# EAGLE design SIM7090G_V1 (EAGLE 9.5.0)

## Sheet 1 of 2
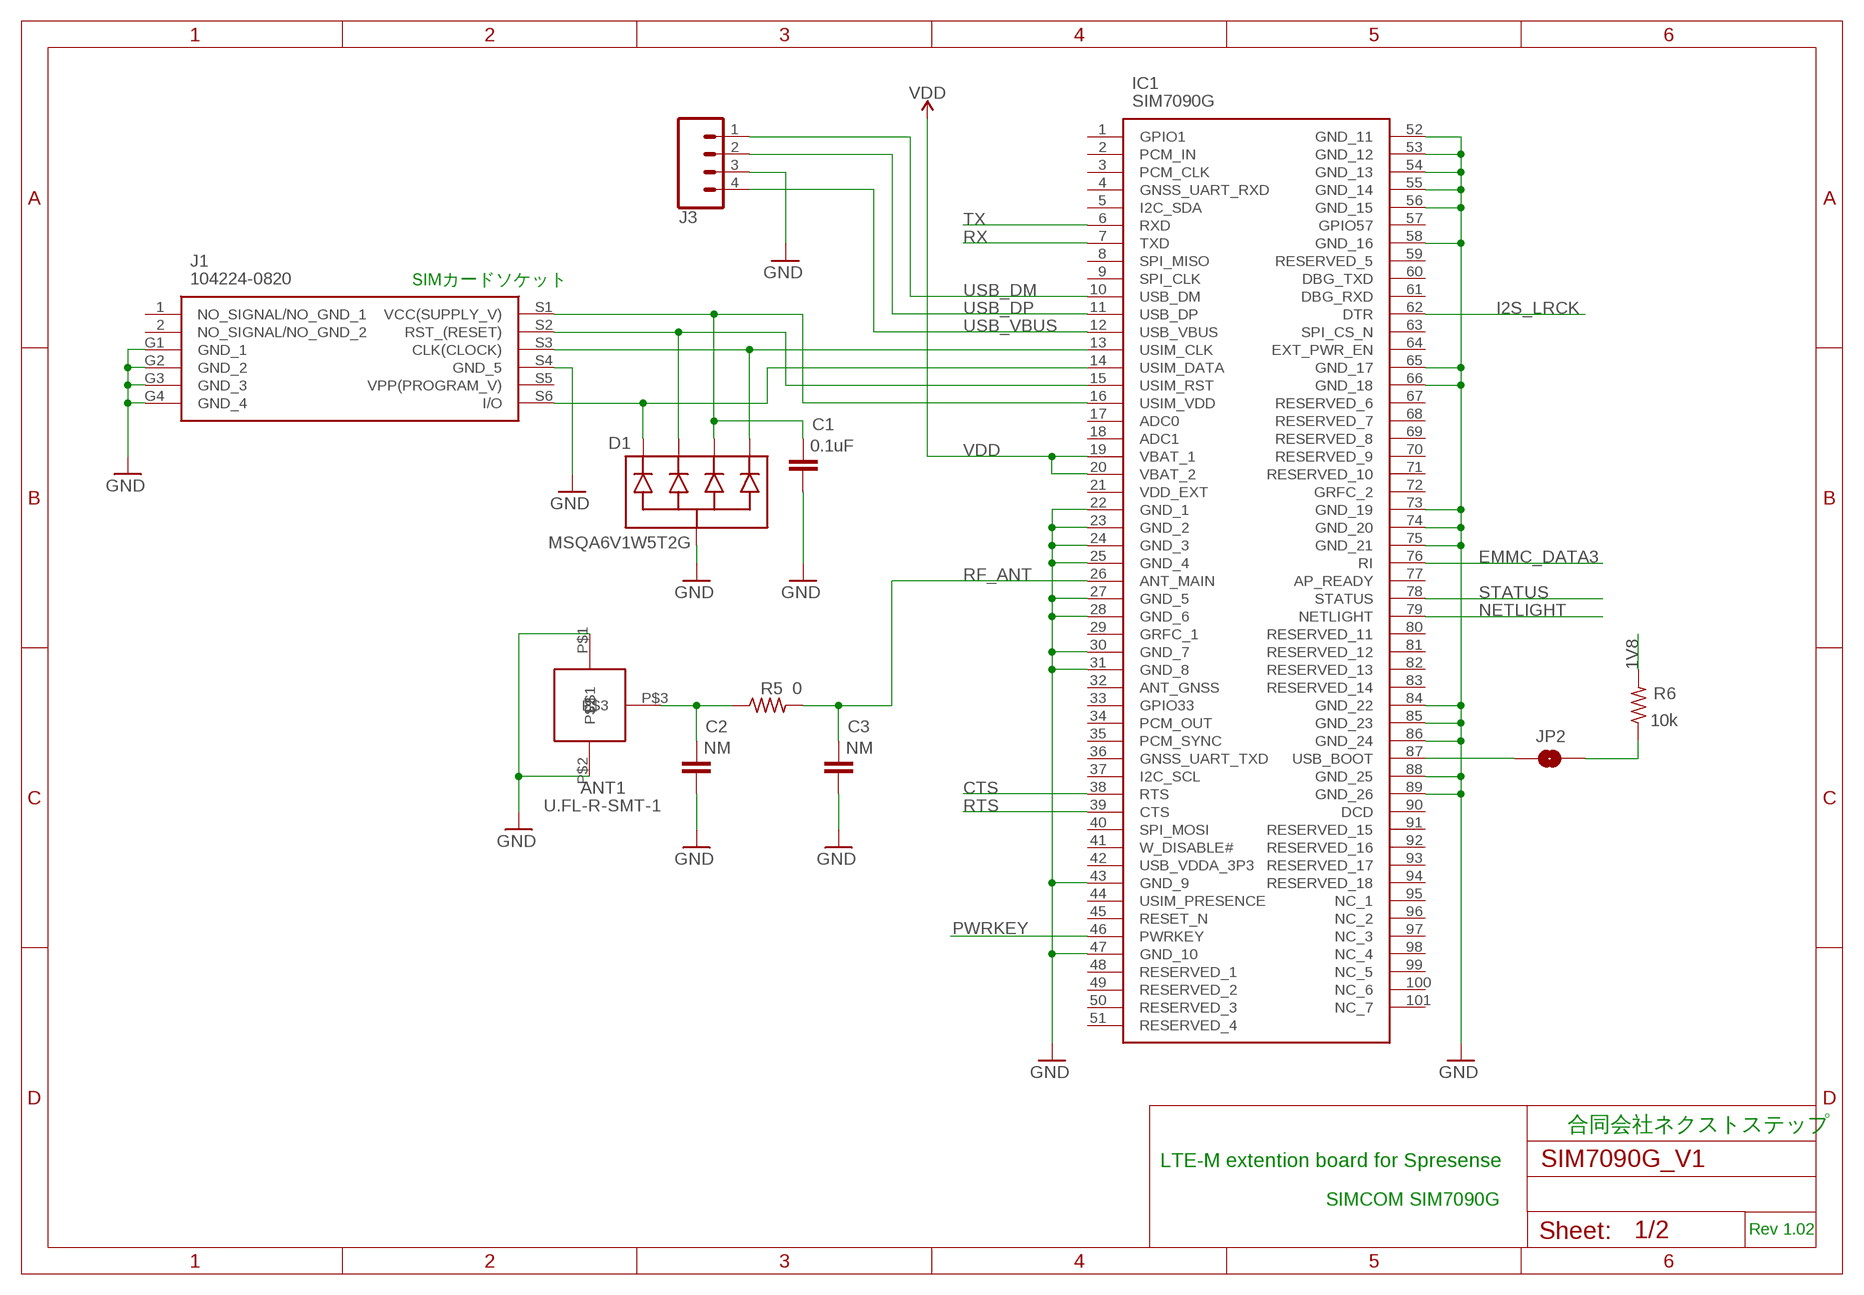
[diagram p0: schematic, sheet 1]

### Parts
ANT1  U.FL-R-SMT-1  [U.FL-R-SMT-1]
C1  0.1uF  C-EUC0603K  [C0603K]
C2  NM  C-EUC0603K  [C0603K]
C3  NM  C-EUC0603K  [C0603K]
D1  MSQA6V1W5T2G  TVS-DIODE-ARRAY-4X  [SOT-353]
IC1  SIM7090G  [SIM7090G]
J1  104224-0820  [1042240820]
J3  CONN_041.27MM  [1X04_1.27MM]
JP2  JUMPER-SMT_2_NO_NO-SILK  [SMT-JUMPER_2_NO_NO-SILK]
R5  0  R-US_R0603  [R0603]
R6  10k  R-US_R0603  [R0603]

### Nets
1V8: R6.2 ; also sheet 2
CTS: IC1.38(RTS) ; also sheet 2
EMMC_DATA3: IC1.76(RI) ; also sheet 2
GND: ANT1.P$1 ANT1.P$2 C1.2 C2.2 C3.2 D1.2(COM) IC1.22(GND_1) IC1.23(GND_2) IC1.24(GND_3) IC1.25(GND_4) IC1.27(GND_5) IC1.28(GND_6) IC1.30(GND_7) IC1.31(GND_8) IC1.43(GND_9) IC1.47(GND_10) IC1.52(GND_11) IC1.53(GND_12) IC1.54(GND_13) IC1.55(GND_14) IC1.56(GND_15) IC1.58(GND_16) IC1.65(GND_17) IC1.66(GND_18) IC1.73(GND_19) IC1.74(GND_20) IC1.75(GND_21) IC1.84(GND_22) IC1.85(GND_23) IC1.86(GND_24) IC1.88(GND_25) IC1.89(GND_26) J1.G1(GND_1) J1.G2(GND_2) J1.G3(GND_3) J1.G4(GND_4) J1.S4(GND_5) J3.3 ; also sheet 2
I2S_LRCK: IC1.62(DTR) ; also sheet 2
N$2: IC1.87(USB_BOOT) JP2.1
N$3: JP2.2 R6.1
N$4: ANT1.P$3 C2.1 R5.1
NETLIGHT: IC1.79(NETLIGHT) ; also sheet 2
PWRKEY: IC1.46(PWRKEY) ; also sheet 2
RF_ANT: C3.1 IC1.26(ANT_MAIN) R5.2
RTS: IC1.39(CTS) ; also sheet 2
RX: IC1.7(TXD) ; also sheet 2
SIM_CLK1: D1.1 IC1.13(USIM_CLK) J1.S3(CLK(CLOCK))
SIM_DATA1: D1.5 IC1.14(USIM_DATA) J1.S6(I/O)
SIM_RST1: D1.4 IC1.15(USIM_RST) J1.S2(RST_(RESET))
SIM_VCC1: C1.1 D1.3 IC1.16(USIM_VDD) J1.S1(VCC(SUPPLY_V))
STATUS: IC1.78(STATUS) ; also sheet 2
TX: IC1.6(RXD) ; also sheet 2
USB_DM: IC1.10(USB_DM) J3.1
USB_DP: IC1.11(USB_DP) J3.2
USB_VBUS: IC1.12(USB_VBUS) J3.4
VDD: IC1.19(VBAT_1) IC1.20(VBAT_2) ; also sheet 2
Unconnected: IC1.1(GPIO1) IC1.2(PCM_IN) IC1.3(PCM_CLK) IC1.4(GNSS_UART_RXD) IC1.5(I2C_SDA) IC1.8(SPI_MISO) IC1.9(SPI_CLK) IC1.17(ADC0) IC1.18(ADC1) IC1.21(VDD_EXT) IC1.29(GRFC_1) IC1.32(ANT_GNSS) IC1.33(GPIO33) IC1.34(PCM_OUT) IC1.35(PCM_SYNC) IC1.36(GNSS_UART_TXD) IC1.37(I2C_SCL) IC1.40(SPI_MOSI) IC1.41(W_DISABLE#) IC1.42(USB_VDDA_3P3) IC1.44(USIM_PRESENCE) IC1.45(RESET_N) IC1.48(RESERVED_1) IC1.49(RESERVED_2) IC1.50(RESERVED_3) IC1.51(RESERVED_4) IC1.57(GPIO57) IC1.59(RESERVED_5) IC1.60(DBG_TXD) IC1.61(DBG_RXD) IC1.63(SPI_CS_N) IC1.64(EXT_PWR_EN) IC1.67(RESERVED_6) IC1.68(RESERVED_7) IC1.69(RESERVED_8) IC1.70(RESERVED_9) IC1.71(RESERVED_10) IC1.72(GRFC_2) IC1.77(AP_READY) IC1.80(RESERVED_11) IC1.81(RESERVED_12) IC1.82(RESERVED_13) IC1.83(RESERVED_14) IC1.90(DCD) IC1.91(RESERVED_15) IC1.92(RESERVED_16) IC1.93(RESERVED_17) IC1.94(RESERVED_18) IC1.95(NC_1) IC1.96(NC_2) IC1.97(NC_3) IC1.98(NC_4) IC1.99(NC_5) IC1.100(NC_6) IC1.101(NC_7) J1.1(NO_SIGNAL/NO_GND_1) J1.2(NO_SIGNAL/NO_GND_2) J1.S5(VPP(PROGRAM_V))

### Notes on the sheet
- SIMカードソケット
- 合同会社ネクストステップ
- LTE-M extention board for Spresense
- SIMCOM SIM7090G
- Rev 1.02

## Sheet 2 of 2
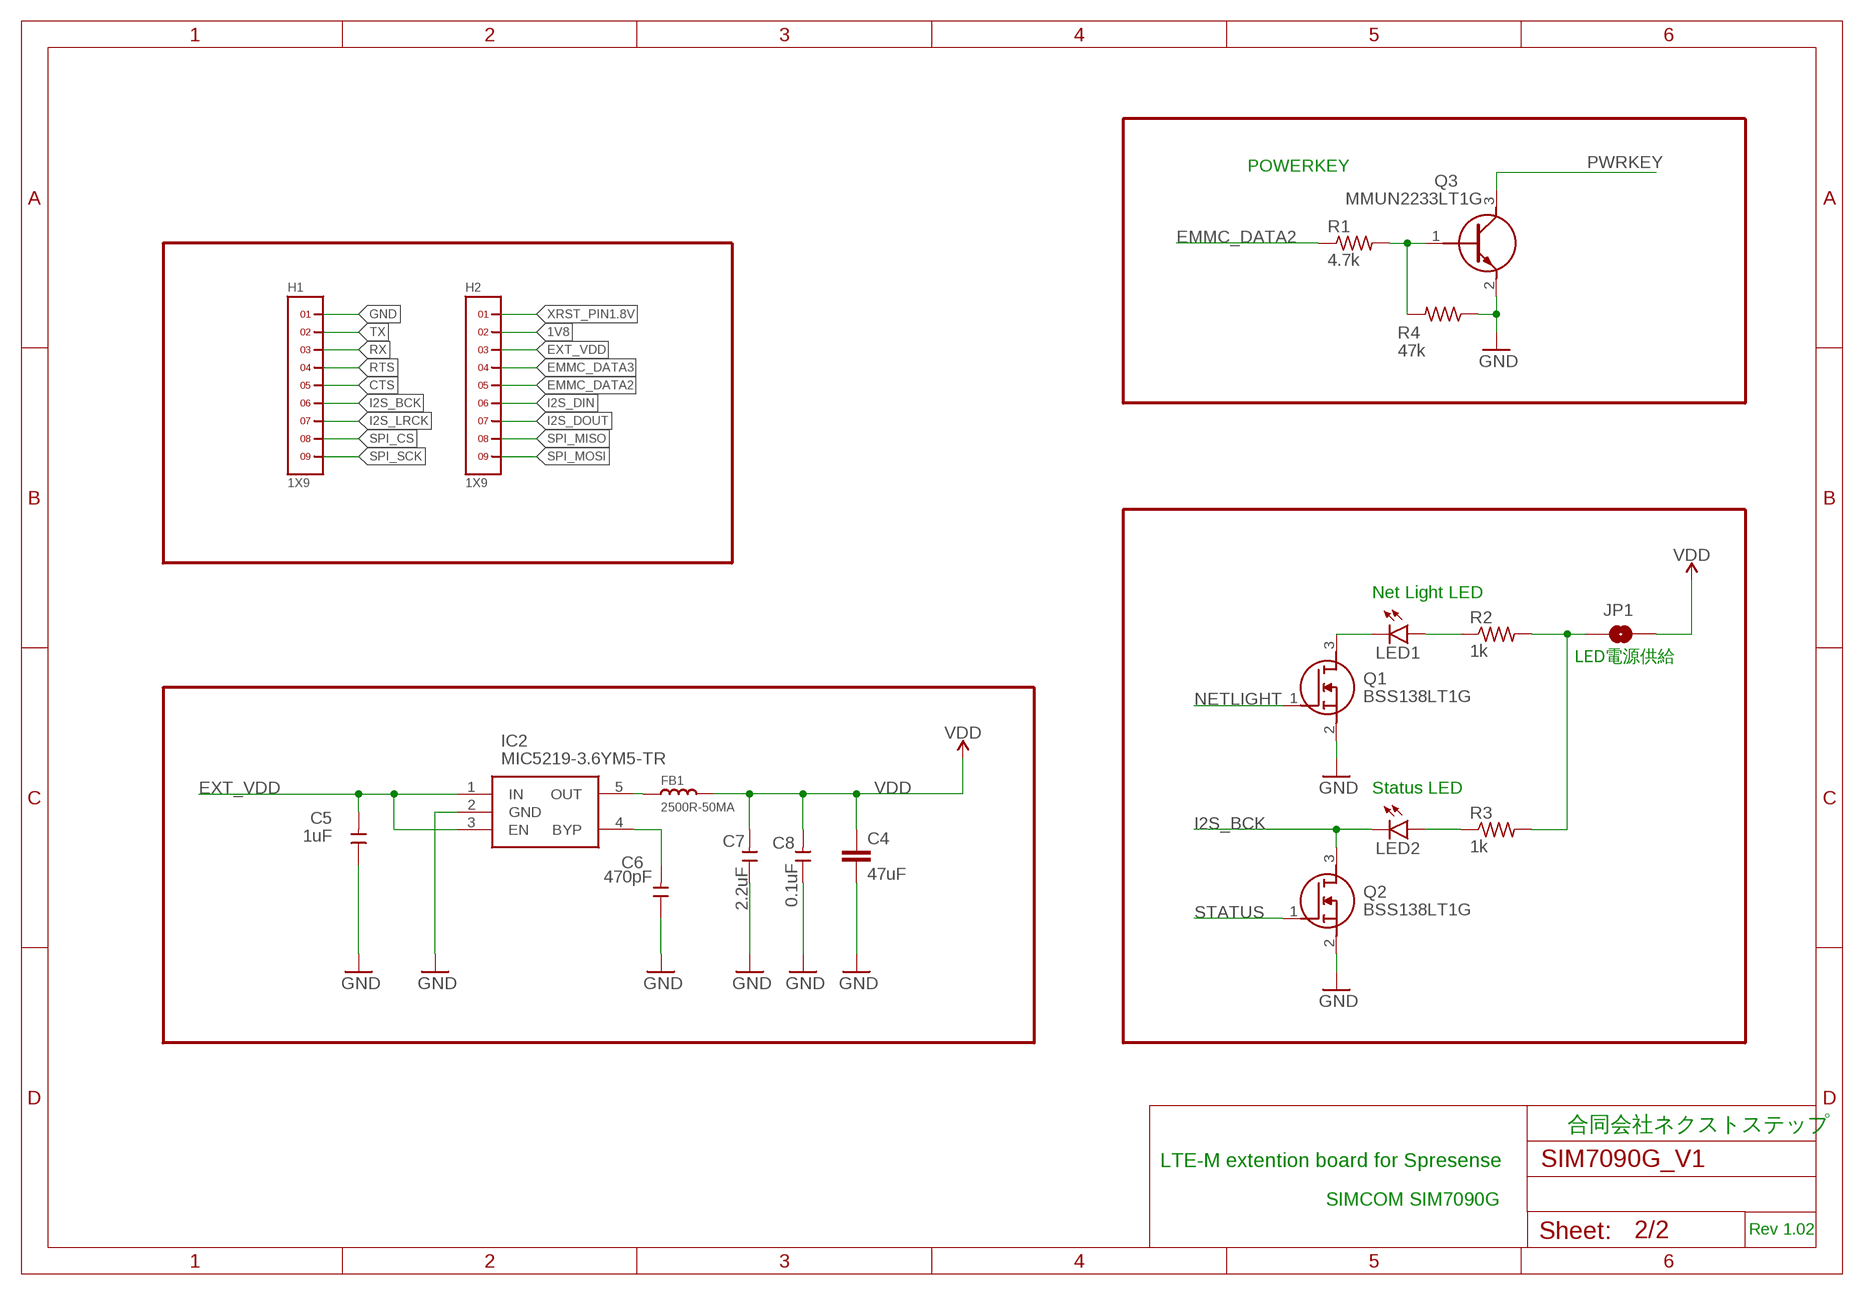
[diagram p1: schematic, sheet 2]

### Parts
C4  47uF  C-EUC0805  [C0805]
C5  1uF  CERAMIC-1UF-25V-10%-X7R(0603)  [C0603]
C6  470pF  CERAMIC-100NF-50V-10%-X7R(0603)  [C0603]
C7  2.2uF  CERAMIC-100NF-50V-10%-X7R(0603)  [C0603]
C8  0.1uF  CERAMIC-100NF-50V-10%-X7R(0603)  [C0603]
FB1  2500R-50MA  SMD-FERRITE-BEAD-2500R-50MA(0603)  [L0603]
H1  1X9  [1X9]
H2  1X9  [1X9]
IC2  MIC5219-3.6YM5-TR  [SOT95P280X145-5N]
JP1  JUMPER-SMT_2_NO_NO-SILK  [SMT-JUMPER_2_NO_NO-SILK]
LED1  LEDCHIP-LED0603  [CHIP-LED0603]
LED2  LEDCHIP-LED0603  [CHIP-LED0603]
Q1  BSS138LT1G  [SOT96P237X111-3N]
Q2  BSS138LT1G  [SOT96P237X111-3N]
Q3  MMUN2233LT1G  [SOT96P237X111-3N]
R1  4.7k  R-US_R0603  [R0603]
R2  1k  R-US_R0603  [R0603]
R3  1k  R-US_R0603  [R0603]
R4  47k  R-US_R0603  [R0603]

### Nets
1V8: H2.2 ; also sheet 1
CTS: H1.5 ; also sheet 1
EMMC_DATA2: H2.5 R1.1
EMMC_DATA3: H2.4 ; also sheet 1
EXT_VDD: C5.2 H2.3 IC2.1(IN) IC2.3(EN)
GND: C4.2 C5.1 C6.1 C7.1 C8.1 H1.1 IC2.2(GND) Q1.2(S) Q2.2(S) Q3.2(E) R4.1 ; also sheet 1
I2S_BCK: H1.6 LED2.C Q2.3(D)
I2S_DIN: H2.6
I2S_DOUT: H2.7
I2S_LRCK: H1.7 ; also sheet 1
N$1: FB1.1 IC2.5(OUT)
N$9: C6.2 IC2.4(BYP)
N$13: JP1.1 R2.2 R3.2
N$16: LED1.A R2.1
N$19: Q3.1(B) R1.2 R4.2
N$22: LED2.A R3.1
NETLIGHT: Q1.1(G) ; also sheet 1
NETLIGHT_MON: LED1.C Q1.3(D)
PWRKEY: Q3.3(C) ; also sheet 1
RTS: H1.4 ; also sheet 1
RX: H1.3 ; also sheet 1
SPI_CS: H1.8
SPI_MISO: H2.8
SPI_MOSI: H2.9
SPI_SCK: H1.9
STATUS: Q2.1(G) ; also sheet 1
TX: H1.2 ; also sheet 1
VDD: C4.1 C7.2 C8.2 FB1.2 JP1.2 ; also sheet 1
XRST_PIN1.8V: H2.1

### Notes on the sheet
- POWERKEY
- Net Light LED
- LED電源供給
- Status LED
- 合同会社ネクストステップ
- LTE-M extention board for Spresense
- SIMCOM SIM7090G
- Rev 1.02

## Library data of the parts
ANT1 = Kris:U.FL-R-SMT-1: U.FL-R-SMT-1
C1-C4 = rcl:C-EU: CAPACITOR, European symbol; SPICEPREFIX: C
C5 = Seeed-Capacitor:CERAMIC-1UF-25V-10%-X7R(0603): 302010139; MPN: CC0603KRX7R8BB105; VALUE: 1uf
C6-C8 = Seeed-Capacitor:CERAMIC-100NF-50V-10%-X7R(0603): 302010138; MPN: CC0603KRX7R9BB104; VALUE: 100nf
D1 = TimWoo-Diodes:TVS-DIODE-ARRAY-4X
FB1 = Seeed-Inductor:SMD-FERRITE-BEAD-2500R-50MA(0603): 303030020
H1 H2 = headers(.1in):1X9
IC1 = SIM7090G:SIM7090G: LPWA Module Source: Datasheet; DESCRIPTION: LPWA Module; HEIGHT: 2.05mm; MANUFACTURER_NAME: Sim Com; MANUFACTURER_PART_NUMBER: SIM7090G
IC2 = SamacSys_Parts:MIC5219-3.6YM5-TR: LDO Voltage Regulators 500mA Peak 1% Low Noise LDO Source: Datasheet; DESCRIPTION: LDO Voltage Regulators 500mA Peak 1% Low Noise LDO; HEIGHT: 1.45mm; MANUFACTURER_NAME: Microchip; MANUFACTURER_PART_NUMBER: MIC5219-3.6YM5-TR; MOUSER_PART_NUMBER: 998-MIC5219-3.6YM5TR; MOUSER_PRICE-STOCK: https://www.mouser.co.uk/ProductDetail/Microchip-Technology-Micrel/MIC5219-36YM5-TR/?qs=U6T8BxXiZAWOHIj15bI33A%3D%3D
J1 = SamacSys_Parts:104224-0820: Memory Card Connectors nanoSIM 1.11mm Card Conn 6Ckt Push/Pull Source: Datasheet; DESCRIPTION: Memory Card Connectors nanoSIM 1.11mm Card Conn 6Ckt Push/Pull; HEIGHT: 1.11mm; MANUFACTURER_NAME: Molex; MANUFACTURER_PART_NUMBER: 104224-0820; MOUSER_PART_NUMBER: 538-104224-0820; MOUSER_PRICE-STOCK: https://www.mouser.com/Search/Refine.aspx?Keyword=538-104224-0820
J3 = SparkFun-Connectors:CONN_04: Multi connection point. Often used as Generic Header-pin footprint for 0.1 inch spaced/style header connections On any of the 0.1 inch spaced packages, you can populate with these: Break Away Headers - Straight (PRT-00116) Break Away Male Headers - Right Angle (PRT-00553) Female Headers (PRT-00115)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
JP1 JP2 = SparkFun-Jumpers:JUMPER-SMT_2_NO: Normally open jumper
LED1 LED2 = led:LED: LED
Q1 Q2 = SamacSys_Parts:BSS138LT1G: MOSFET N-Channel 50V 0.2A SOT23 ON Semiconductor BSS138LT1G N-channel MOSFET Transistor, 0.2 A, 50 V, 3-Pin SOT-23 Source: Datasheet; DESCRIPTION: MOSFET N-Channel 50V 0.2A SOT23 ON Semiconductor BSS138LT1G N-channel MOSFET Transistor, 0.2 A, 50 V, 3-Pin SOT-23; HEIGHT: 1.11mm; MANUFACTURER_NAME: ON Semiconductor; MANUFACTURER_PART_NUMBER: BSS138LT1G; MOUSER_PART_NUMBER: 863-BSS138LT1G; MOUSER_PRICE-STOCK: https://www.mouser.com/Search/Refine.aspx?Keyword=863-BSS138LT1G
Q3 = SamacSys_Parts:MMUN2233LT1G: ON SEMICONDUCTOR - MMUN2233LT1G - TRANSISTOR, SMD NPN Source: Datasheet; DESCRIPTION: ON SEMICONDUCTOR - MMUN2233LT1G - TRANSISTOR, SMD NPN; HEIGHT: 1.11mm; MANUFACTURER_NAME: ON Semiconductor; MANUFACTURER_PART_NUMBER: MMUN2233LT1G; MOUSER_PART_NUMBER: 863-MMUN2233LT1G; MOUSER_PRICE-STOCK: https://www.mouser.com/Search/Refine.aspx?Keyword=863-MMUN2233LT1G
R1-R6 = rcl:R-US_: RESISTOR, American symbol; SPICEPREFIX: R

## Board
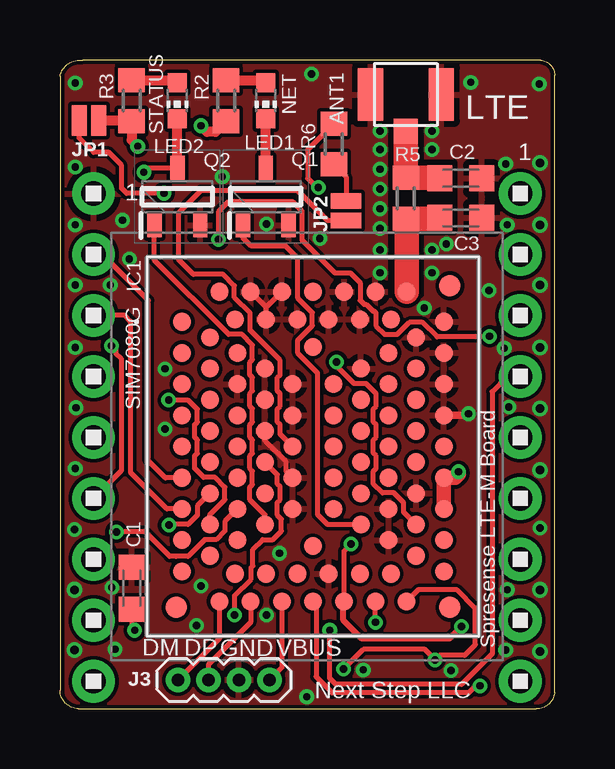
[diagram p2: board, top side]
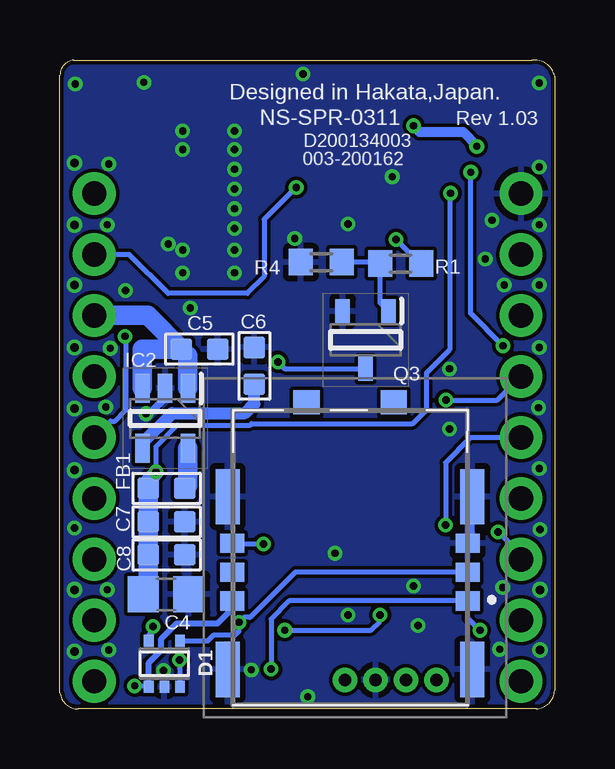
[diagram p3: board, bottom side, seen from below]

Size 20.61 x 27.03 mm. Coordinates in mm from the lower left corner, seen from the top.
Outline: 0,26.35 arc-88 0.95,27.02 20.03,27.02 arc-88 20.61,26.38 20.61,0.67 arc-88 19.84,0 0.76,0 arc-88 0,0.76 0,26.35
Copper layers (1*16): Top 0.035mm / dielectric 1.5mm / Bottom 0.035mm
Design rules "SeeedStudio_2layer_DRU_no_angle_20140221 *": minimum track width 6mil, minimum drill 12mil, track to track 6mil, track to pad 6mil, pad to pad 6mil, via to via 6mil, smd to smd 0mil, copper to edge 6mil, drill to drill 8mil, minimum pad ring 10mil, minimum via ring 6mil, stop-mask expansion 2mil, vias tented up to drill 100mil, thermal gap 10mil
tRestrict: 13 lines

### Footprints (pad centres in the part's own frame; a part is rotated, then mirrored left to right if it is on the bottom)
U.FL-R-SMT-1 = smd 1.05 x 2.2: P$1 -1.475,0; P$2 1.475,0 | smd 1 x 1.05: P$3 0,-1.525
C0603K = smd 1.05 x 1.08: 1 -0.875,0; 2 0.875,0
C0805 = smd 1.3 x 1.5: 1 -0.95,0; 2 0.95,0
C0603 = smd 0.889 x 0.889: 1 0,0.762; 2 0,-0.762
SOT-353 = smd 0.4 x 0.5: 1 -0.65,-0.95; 2 0,-0.95; 3 0.65,-0.95; 4 0.65,0.95; 5 -0.65,0.95
L0603 = smd 0.889 x 0.889: 1 -0.762,0; 2 0.762,0
1X9 = drill 1.016 pad 1.778: 1 0,0; 2 2.54,0; 3 5.08,0; 4 7.62,0; 5 10.16,0; 6 12.7,0; 7 15.24,0; 8 17.78,0; 9 20.32,0
SIM7090G = smd 0.75 x 0.75: 1 -5.45,5.2; 2 -5.45,3.9; 3 -5.45,2.6; 4 -5.45,1.3; 5 -5.45,0; 6 -5.45,-1.3; 7 -5.45,-2.6; 8 -5.45,-3.9; 9 -5.45,-5.2; 10 -3.9,-6.45; 11 -2.6,-6.45; 12 -1.3,-6.45; 13 0,-6.45; 14 1.3,-6.45; 15 2.6,-6.45; 16 3.9,-6.45; 17 5.45,-5.2; 18 5.45,-3.9; 19 5.45,-2.6; 20 5.45,-1.3; 21 5.45,0; 22 5.45,1.3; 23 5.45,2.6; 24 5.45,3.9; 25 5.45,5.2; 26 3.9,6.45; 27 2.6,6.45; 28 1.3,6.45; 29 0,6.45; 30 -1.3,6.45; 31 -2.6,6.45; 32 -3.9,6.45; 33 -4.3,4.55; 34 -4.3,3.25; 35 -4.3,1.95; 36 -4.3,0.65; 37 -4.3,-0.65; 38 -4.3,-1.95; 39 -4.3,-3.25; 40 -4.3,-4.55; 41 -1.95,-5.3; 42 -0.65,-5.3; 43 0.65,-5.3; 44 1.95,-5.3; 45 4.3,-4.55; 46 4.3,-3.25; 47 4.3,-1.95; 48 4.3,-0.65; 49 4.3,0.65; 50 4.3,1.95; 51 4.3,3.25; 52 4.3,4.55; 53 1.95,5.3; 54 0.65,5.3; 55 -0.65,5.3; 56 -1.95,5.3; 57 -3.15,3.9; 58 -3.15,2.6; 59 -3.15,1.3; 60 -3.15,0; 61 -3.15,-1.3; 62 -3.15,-2.6; 63 -3.15,-3.9; 64 0,-4.15; 65 3.15,-3.9; 66 3.15,-2.6; 67 3.15,-1.3; 68 3.15,0; 69 3.15,1.3; 70 3.15,2.6; 71 3.15,3.9; 72 0,4.15; 73 -2,3.25; 74 -2,1.95; 75 -2,0.65; 76 -2,-0.65; 77 -2,-1.95; 78 -2,-3.25; 79 2,-3.25; 80 2,-1.95; 81 2,-0.65; 82 2,0.65; 83 2,1.95; 84 2,3.25; 85 -0.85,2.6; 86 -0.85,1.3; 87 -0.85,0; 88 -0.85,-1.3; 89 -0.85,-2.6; 90 0.85,-2.6; 91 0.85,-1.3; 92 0.85,0; 93 0.85,1.3; 94 0.85,2.6; 95 -3.25,5.3; 96 -3.25,-5.3; 97 3.25,-5.3; 98 3.25,5.3 | smd 0.9 x 0.9: 99 -5.7,-6.7; 100 5.7,-6.7; 101 5.7,6.7
SOT95P280X145-5N = smd 1.2 x 0.6: 1 -1.25,0.95; 2 -1.25,0; 3 -1.25,-0.95; 4 1.25,-0.95; 5 1.25,0.95
1042240820 = smd 1.1 x 1: 1 -2.02,6.063; 2 1.62,6.063 | smd 1 x 2.3: G1 -5.3,-5.063; G2 -5.3,2.137; G3 4.9,2.137; G4 4.9,-5.063 | smd 1 x 0.8: S1 4.7,-2.212; S2 4.7,-1.012; S3 -5.1,-2.212; S4 4.7,0.188; S5 -5.1,-1.012; S6 -5.1,0.188
1X04_1.27MM = drill 0.508 pad 1: 1 0,0; 2 1.27,0; 3 2.54,0; 4 3.81,0
SMT-JUMPER_2_NO_NO-SILK = smd 0.635 x 1.27: 1 -0.406,0; 2 0.406,0
CHIP-LED0603 = smd 0.8 x 0.8: A 0,-0.75; C 0,0.75
SOT96P237X111-3N = smd 1 x 0.6: 1 -1.2,0.955; 2 -1.2,-0.955; 3 1.2,0
R0603 = smd 1 x 1.1: 1 -0.85,0; 2 0.85,0

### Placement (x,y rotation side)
ANT1  14.41,25.59 0 top
C1  2.98,5.02 90 top
C2  16.7,22.1 0 top
C3  16.7,20.45 0 top
C4  16.19,4.76 0 bottom
C5  14.8,14.99 270 bottom
C6  12.51,14.29 0 bottom
C7  16.16,7.78 270 bottom
C8  16.16,6.41 270 bottom
D1  16.26,1.87 0 bottom
FB1  16.16,9.18 180 bottom
H1  1.4,21.46 270 top
H2  19.18,21.46 270 top
IC1  10.54,10.92 0 top
IC2  16.22,12.1 270 bottom
J1  8.32,6.7 0 bottom
J3  4.92,1.2 0 top
JP1  1.21,24.51 180 top
JP2  11.93,20.75 90 top
LED1  8.57,25.34 180 top
LED2  4.89,25.34 180 top
Q1  8.57,21.34 90 top
Q2  4.89,21.34 90 top
Q3  7.87,15.37 270 bottom
R1  6.41,18.54 180 bottom
R2  6.92,25.34 270 top
R3  2.98,25.34 270 top
R4  9.72,18.61 0 bottom
R5  14.41,21.27 270 top
R6  11.41,23.53 90 top

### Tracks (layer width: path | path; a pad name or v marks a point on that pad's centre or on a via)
1V8  (via drill 0.3)
  Top 0.203: R6.2 10.32,23.28 10.32,22.1 10.7,21.72 v10.76,21.72
  Bottom 0.203: v10.76,21.72 12.1,20.38 12.1,18 12.79,17.3 16.1,17.3 17.72,18.92 H2.2
CTS  (via drill 0.3)
  Top 0.203: IC1.38 5.72,8.45 5.72,8.06 5.34,7.68 4.57,7.68 v4.54,7.65
  Bottom 0.203: v4.54,7.65 4.54,10.25 3.49,11.3 H1.5
EMMC_DATA2  (via drill 0.3)
  Top 0.203: v17.9,15.51 17.88,15.49 15.71,15.49 15.1,16.1 14.56,16.1 14.05,15.59 13.53,15.59 13.16,15.96 13.16,16.49 13.08,16.57 13.03,16.57 12.75,16.85 12.68,16.85 12.51,17.02 12.51,17.75 12.1,18.16 11.45,18.16 10.08,19.53 10.08,20.74 9.71,21.11 7.02,21.11 6.6,20.7 v6.6,19.55
  Bottom 0.203: H2.5 18.5,11.98 18.31,11.98 17.87,12.43 17.87,15.48 v17.9,15.51 | v6.6,19.55 5.6,18.54 R1.1
EMMC_DATA3  (via drill 0.3)
  Top 0.203: H2.4 18.64,13.84 18,13.21 18,2.29 16.73,1.02 11.49,1.02 11.24,1.27 v11.24,3.27 | v7.27,3.91 7.27,4.71 7.96,5.4 7.96,5.88 8.03,5.95 8.03,6.64 8.44,7.04 8.86,7.04 9.22,7.4 9.22,7.9 9.06,8.06 9.06,8.6 9.17,8.71 9.17,9.25 9.06,9.36 9.06,9.75 IC1.76
  Bottom 0.203: v11.24,3.27 7.65,3.27 7.27,3.65 v7.27,3.91
EXT_VDD
  Bottom 0.813: C5.2 16.95,16.38 H2.3 | IC2.3 17.17,14.99 C5.2 | C5.2 15.27,14.7 IC2.1
GND  (via drill 0.3, 0.35)
  Top 0.203: IC1.88 9.42,9.89 9.42,10.29 8.54,11.16 IC1.75 | 8.59,16.72 IC1.30 | IC1.56 8.59,16.72 | 8.59,16.72 IC1.31
  Top 0.305: v17.02,12.29 16.95,12.22 IC1.22
  Bottom 0.203: J1.S4 3.42,7.09 J1.G3
  Bottom 0.305: IC2.2 16.22,12.95 16.89,12.29 v17.02,12.29
  other vias: 15.18,16.7 17.88,17.43 16.29,1.59 4.38,14.16 9.14,6.48 10.28,0.5 12.64,1.62 18.57,2.44 18.64,4.95 20,7.52 18.7,12.57 18.51,15.02 13.34,18.16 13.34,19.11 13.34,20 13.34,20.83 13.34,21.65 13.34,22.48 13.34,23.3 13.34,24.07 15.49,24.07 15.49,23.3 15.49,18.16 15.49,19.11 16.1,19.37 18.64,20.16 18.57,22.7 17.11,26.1 19.97,26.04 0.63,26.07 10.48,26.45 6.76,22.16 10.83,19.59 8.6,20.19 2.6,20.35 0.63,22.57 2.89,18.73 2.1,17.65 5.87,5.11 8.6,3.91 5.68,3.46 2.29,2.48 2.16,5.05 0.63,15.05 0.67,12.54 0.63,10 4.38,11.65 0.6,7.46 0.63,17.65 0.63,20.16 20,2.38 20,4.95 20,9.94 20,12.51 20,15.05 20,17.65 20,20.16 20,22.73 0.6,4.95 0.6,2.44
  pour Top: 0,27.02 20.64,27.02 20.64,-0.19 0,-0.19
  pour Bottom: 0,27.02 20.64,27.02 20.64,-0.13 0,-0.13
I2S_BCK  (via drill 0.3)
  Top 0.203: H1.6 2.55,9.92 2.55,14.57 2.33,14.79 2.33,15.12 v2.15,15.12 | v3.49,22.35 3.68,22.54 Q2.3
  Top 0.406: Q2.3 LED2.C
  Bottom 0.203: v2.15,15.12 3.49,16.47 v3.49,22.35
I2S_LRCK  (via drill 0.3)
  Top 0.203: IC1.62 6.87,7.8 6.87,7.41 6.5,7.04 6.02,7.04 5.61,6.63 5.33,6.35 4.83,6.35 4.57,6.35 3.56,7.37 v2.35,7.37
  Bottom 0.203: v2.35,7.37 1.4,6.41 H1.7
N$1
  Bottom 0.813: FB1.1 15.27,9.3 IC2.5
N$2
  Top 0.203: IC1.87 9.17,11.44 9.17,11.83 9.06,11.94 9.06,12.5 9.17,12.61 9.17,13.13 9.06,13.24 9.06,13.8 9.17,13.91 9.17,14.51 7.92,15.76 7.92,16.48 7.27,17.13 7.27,17.63 6.8,18.1 5.56,18.1 4.95,18.7 4.95,20.67 5.88,21.6 9.89,21.6 11.15,20.35 JP2.1
N$3
  Top 0.203: R6.1 11.93,22.16 JP2.2
N$4
  Top 1.025: ANT1.P$3 R5.1 15.8,22.12 C2.1
N$9
  Bottom 0.508: C6.2 12.51,12.7 12.89,12.32 15.94,12.32 17.17,11.08 IC2.4
N$13  (via drill 0.3)
  Top 0.406: JP1.1 2.96,24.51 R3.2 2.98,23.69 v3.24,23.43 | R2.2 6.47,24.04 6.13,24.04 v5.87,24.29
  Bottom 0.406: v5.87,24.29 5.62,24.04 3.81,24.04 3.24,23.46 v3.24,23.43
N$16
  Top 0.406: R2.1 8.47,26.19 LED1.A
N$19
  Bottom 0.203: R4.2 7.33,18.61 R1.2 7.26,16.91 Q3.1
N$22
  Top 0.406: R3.1 4.79,26.19 LED2.A
NETLIGHT
  Top 0.203: IC1.79 11.15,7.67 10.74,8.08 10.74,13.98 9.91,14.81 9.91,15.35 10.52,15.96 10.52,16.5 9.91,17.11 9.91,17.14 9.91,18.75 9.91,18.76 9.4,19.27 7.97,19.27 7.62,19.62 Q1.1
NETLIGHT_MON
  Top 0.406: Q1.3 LED1.C
PWRKEY  (via drill 0.3)
  Top 0.203: IC1.46 14.32,8.19 14.32,8.58 13.91,8.99 13.43,8.99 13.06,9.36 13.06,9.9 13.17,10.01 13.17,10.53 13.06,10.64 13.06,11.2 13.17,11.31 13.17,11.83 13.06,11.94 13.06,12.5 13.17,12.61 13.17,13.13 12.76,13.54 12.26,13.54 11.52,14.28 v11.52,14.45
  Bottom 0.203: v11.52,14.45 11.24,14.17 Q3.3
RF_ANT
  Top 1.025: IC1.26 14.44,20.4 R5.2 15.8,20.42 C3.1
RTS  (via drill 0.3)
  Top 0.203: IC1.39 6.24,8.08 6.87,8.71 6.87,9.23 6.46,9.64 5.98,9.64 5.61,10.01 5.61,10.53 5.72,10.64 5.72,11.2 5.61,11.31 5.61,11.83 5.72,11.94 5.72,12.48 5.35,12.85 4.54,12.85 v4.53,12.86
  Bottom 0.203: v4.53,12.86 2.38,12.86 H1.4
RX
  Top 0.203: IC1.7 4.46,8.32 2.95,9.82 2.95,16.13 2.7,16.38 H1.3
SIM_CLK1  (via drill 0.3)
  Top 0.203: v17.49,0.95 17.33,0.95 17.04,0.66 11.34,0.66 10.67,1.33 10.67,4.35 IC1.13
  Bottom 0.203: v17.49,0.95 16.93,0.95 D1.1
  Bottom 0.254: D1.1 16.91,1.92 16.38,2.45 16.38,2.92 15.75,3.56 14.03,3.56 13.42,4.17 J1.S3
SIM_DATA1  (via drill 0.3)
  Top 0.203: IC1.14 11.84,6.57 v12.13,6.86
  Top 0.254: v16.73,3.43 16.22,2.92 12.57,2.92 11.81,3.68 11.81,4.44 IC1.14
  Bottom 0.203: v12.13,6.86 13.39,6.86 J1.S6
  Bottom 0.254: v16.73,3.43 16.73,3.21 16.91,3.03 D1.5
SIM_RST1  (via drill 0.3)
  Top 0.203: v13.14,3.6 IC1.15
  Bottom 0.203: D1.4 14.45,2.82 14.19,3.08 13.3,3.08 13.14,3.24 v13.14,3.6 12.94,3.8 12.69,3.8 10.8,5.69 J1.S2
SIM_VCC1  (via drill 0.3)
  Top 0.203: IC1.16 14.92,4.95 16.54,4.95 17.3,4.19 17.3,2.67 16.86,2.22 15.81,2.22 v15.62,2.03 15.62,2.06 15.21,2.48 12.64,2.48 v11.81,1.65 | C1.1 2.98,3.4 v3.11,3.27
  Bottom 0.203: v15.62,2.03 15.62,1.68 15.61,1.67 D1.3 | v11.81,1.65 11.81,3.75 11.07,4.49 J1.S1 3.62,3.78 v3.11,3.27
STATUS
  Top 0.203: IC1.78 8.54,8.08 7.91,8.71 7.91,9.23 8.02,9.34 8.02,9.9 7.91,10.01 7.91,10.53 8.02,10.64 8.02,11.2 7.91,11.31 7.91,11.83 8.02,11.94 8.02,12.5 7.91,12.61 7.91,13.13 8.02,13.24 8.02,13.8 7.91,13.91 7.91,14.43 8.02,14.54 8.02,15.16 7.58,15.59 7.03,15.59 3.94,18.69 Q2.1
TX
  Top 0.203: IC1.6 4.39,9.62 3.68,10.33 3.68,17.02 1.78,18.92 H1.2
USB_DM
  Top 0.203: IC1.10 6.64,2.92 J3.1
USB_DP
  Top 0.203: IC1.11 7.94,3.59 6.19,1.84 J3.2
USB_VBUS
  Top 0.203: IC1.12 9.24,1.71 J3.4
VDD  (via drill 0.3)
  Top 0.203: v4.33,21.48 2.77,21.48 2.57,21.68 2.57,22.64 2.03,23.18 1.4,23.18 0.8,23.77 JP1.2
  Top 0.61: IC1.19 IC1.20 16.47,9.62 16.61,9.76 v16.61,9.87
  Bottom 0.203: v16.61,9.87 16.61,10.92 15.72,11.81 12.68,11.81 12.62,11.88 5.91,11.88 5.33,12.45 5.33,14 4.38,14.96 4.38,21.48 v4.33,21.48
  Bottom 0.61: v16.61,9.87 16.61,9.84 16.92,9.52 FB1.2
  Bottom 0.813: FB1.2 C7.2 C8.2 16.92,4.98 C4.1

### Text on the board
tPlace: NET | LTE | STATUS | 1 | 1 | SIM7080G | Spresense LTE-M Board | DM | DP | GND | VBUS | Next Step LLC
bPlace: Designed in Hakata,Japan. | Rev 1.03 | NS-SPR-0311 | D200134003 | 003-200162

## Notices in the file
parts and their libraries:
SparkFun-Jumpers: Licensing: Creative Commons ShareAlike 4.0 International - https://creativecommons.org/licenses/by-sa/4.0
